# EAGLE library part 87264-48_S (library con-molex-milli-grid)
RECEPTACAL
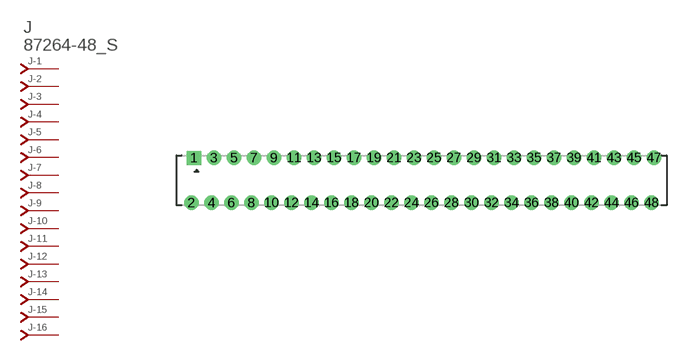
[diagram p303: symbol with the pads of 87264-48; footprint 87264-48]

Designator prefix J; gates -1=J-NV -2=J-N -3=J-N -4=J-N -5=J-N -6=J-N -7=J-N -8=J-N -9=J-N -10=J-N -11=J-N -12=J-N -13=J-N -14=J-N -15=J-N -16=J-N -17=J-N -18=J-N -19=J-N -20=J-N -21=J-N -22=J-N -23=J-N -24=J-N -25=J-N -26=J-N -27=J-N -28=J-N -29=J-N -30=J-N -31=J-N -32=J-N -33=J-N -34=J-N -35=J-N -36=J-N -37=J-N -38=J-N -39=J-N -40=J-N -41=J-N -42=J-N -43=J-N -44=J-N -45=J-N -46=J-N -47=J-N -48=J-N

## 87264-48_S  [87264-48]
1  -1:J  pas
2  -2:J  pas
3  -3:J  pas
4  -4:J  pas
5  -5:J  pas
6  -6:J  pas
7  -7:J  pas
8  -8:J  pas
9  -9:J  pas
10  -10:J  pas
11  -11:J  pas
12  -12:J  pas
13  -13:J  pas
14  -14:J  pas
15  -15:J  pas
16  -16:J  pas
17  -17:J  pas
18  -18:J  pas
19  -19:J  pas
20  -20:J  pas
21  -21:J  pas
22  -22:J  pas
23  -23:J  pas
24  -24:J  pas
25  -25:J  pas
26  -26:J  pas
27  -27:J  pas
28  -28:J  pas
29  -29:J  pas
30  -30:J  pas
31  -31:J  pas
32  -32:J  pas
33  -33:J  pas
34  -34:J  pas
35  -35:J  pas
36  -36:J  pas
37  -37:J  pas
38  -38:J  pas
39  -39:J  pas
40  -40:J  pas
41  -41:J  pas
42  -42:J  pas
43  -43:J  pas
44  -44:J  pas
45  -45:J  pas
46  -46:J  pas
47  -47:J  pas
48  -48:J  pas

## Footprint 87264-48 (pad centres in mm)
RECEPTACAL Dual Row, Side Entry
drill 0.914 square: 1 -22.75,2.25
drill 0.914: 2 -23,-2.25; 3 -20.75,2.25; 4 -21,-2.25; 5 -18.75,2.25; 6 -19,-2.25; 7 -16.75,2.25; 8 -17,-2.25; 9 -14.75,2.25; 10 -15,-2.25; 11 -12.75,2.25; 12 -13,-2.25; 13 -10.75,2.25; 14 -11,-2.25; 15 -8.75,2.25; 16 -9,-2.25; 17 -6.75,2.25; 18 -7,-2.25; 19 -4.75,2.25; 20 -5,-2.25; 21 -2.75,2.25; 22 -3,-2.25; 23 -0.75,2.25; 24 -1,-2.25; 25 1.25,2.25; 26 1,-2.25; 27 3.25,2.25; 28 3,-2.25; 29 5.25,2.25; 30 5,-2.25; 31 7.25,2.25; 32 7,-2.25; 33 9.25,2.25; 34 9,-2.25; 35 11.25,2.25; 36 11,-2.25; 37 13.25,2.25; 38 13,-2.25; 39 15.25,2.25; 40 15,-2.25; 41 17.25,2.25; 42 17,-2.25; 43 19.25,2.25; 44 19,-2.25; 45 21.25,2.25; 46 21,-2.25; 47 23.25,2.25; 48 23,-2.25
